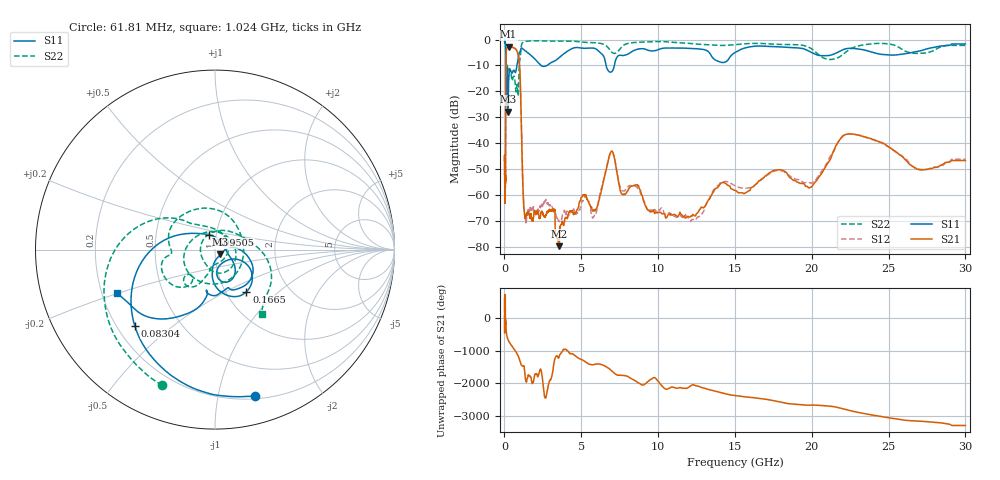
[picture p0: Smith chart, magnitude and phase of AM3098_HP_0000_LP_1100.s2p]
! Date/Time: Thu, Feb 28, 2019 8:31 AM
! Network Analyzer: Agilent Technologies E8364B Rev: A.07.50.67
! Sweep from 0.010 to 30.000 GHz, 1601 Points, Sweep Type: LOG
! Power Supply: 5.023 V, 0.002 A
# Hz S DB R 50
!freq MagS11 AngS11 MagS21 AngS21 MagS12 AngS12 MagS22 AngS22
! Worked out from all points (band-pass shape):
!   1601 points, 10 MHz to 30 GHz, reference 50 ohm
!   highest |S21| = -2.78 dB at 266.5 MHz (marker M1); lowest = -79.8 dB at 3.577 GHz (marker M2)
!   |S21| within 3 dB of the highest: 104.5 MHz to 887.5 MHz (782.9 MHz wide, 158 % of centre)
!   lowest |S11| = -27.9 dB at 232.8 MHz (marker M3), VSWR 1.08, Z = 53 - j2.86 ohm
!   |S11| at or under -10 dB: 90.4 MHz to 811.2 MHz (720.8 MHz wide, 160 % of centre); 2.375 GHz to 2.771 GHz (396.2 MHz wide, 15.4 % of centre); 6.616 GHz to 7.154 GHz (538.4 MHz wide, 7.82 % of centre)
!   |S22| runs from -22.9 to -0.5 dB; largest |S21 - S12| = 0.01
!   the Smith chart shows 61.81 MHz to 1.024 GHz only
!   S11 on the Smith chart (normalised r, x): 61.81 MHz: 0.22, -1.29; 83.04 MHz: 0.27, -0.37; 95.05 MHz: 0.92, +0.15; 166.5 MHz: 1.24, -0.64; 1.024 GHz: 0.26, -0.20
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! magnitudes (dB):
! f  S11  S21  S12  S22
! 10 MHz  -0.3  -46.8  -45.1  -0.6
! 38.04 MHz  -0.5  -62.9  -59.4  -1.0
! 61.81 MHz  -1.5  -54.2  -55.5  -1.8
! 83.04 MHz  -4.2  -30.0  -30.1  -4.7
! 95.05 MHz  -21.0  -9.8  -9.8  -22.4
! 144.7 MHz  -14.5  -3.4  -3.4  -12.6
! 166.5 MHz  -10.7  -3.3  -3.3  -10.1
! 232.8 MHz  -27.9  -2.8  -2.8  -12.1
! 266.5 MHz  -17.1  -2.8  -2.7  -12.3
! 550.5 MHz  -12.3  -3.1  -3.0  -14.9
! 885.5 MHz  -7.7  -5.7  -5.7  -21.7
! 1.024 GHz  -4.5  -14.8  -14.8  -7.0
! 1.321 GHz  -4.2  -68.1  -68.1  -0.8
! 2.084 GHz  -8.2  -66.9  -65.9  -0.5
! 3.577 GHz  -6.9  -79.8  -70.4  -0.6
! 5.87 GHz  -3.4  -66.2  -67.8  -1.2
! 6.924 GHz  -12.6  -43.4  -43.5  -4.4
! 7.926 GHz  -5.9  -59.4  -57.8  -1.7
! 12.31 GHz  -3.5  -67.7  -69.5  -1.6
! 19.9 GHz  -4.7  -57.1  -55.3  -3.3
! 22.67 GHz  -3.4  -36.5  -36.6  -3.2
! 30 GHz  -1.7  -46.7  -46.2  -2.3
